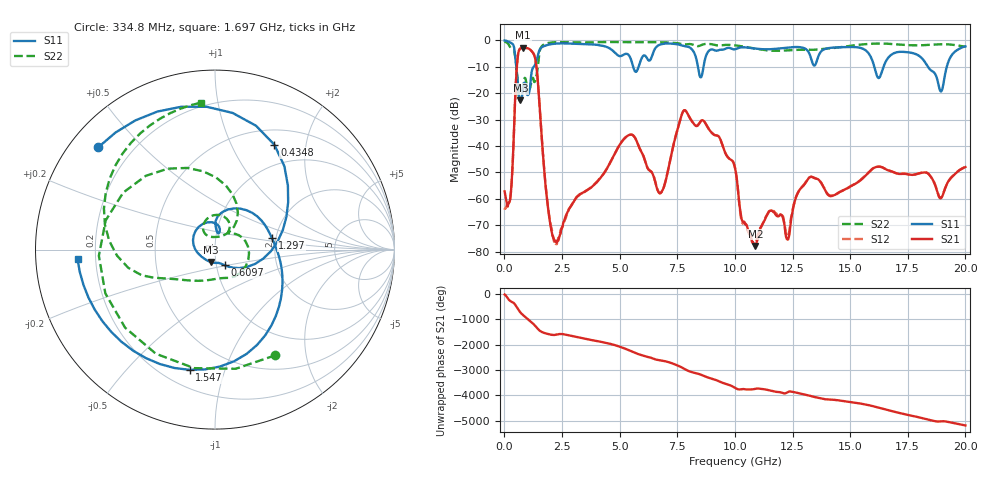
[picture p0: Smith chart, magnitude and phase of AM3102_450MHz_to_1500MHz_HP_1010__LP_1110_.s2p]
!Agilent Technologies,E8364B,MY43040894,A.07.50.67
!Agilent E8364B: A.07.50.67
!Date: Thursday, January 11, 2018 06:21:26
!Correction: S11(Full 2 Port(1,2))
!S21(Full 2 Port(1,2))
!S12(Full 2 Port(1,2))
!S22(Full 2 Port(1,2))
!S2P File: Measurements: S11, S21, S12, S22:
# Hz S  dB  R 50
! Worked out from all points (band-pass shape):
!   1601 points, 10 MHz to 20 GHz, reference 50 ohm
!   highest |S21| = -2.85 dB at 809.6 MHz (marker M1); lowest = -77.8 dB at 10.89 GHz (marker M2)
!   |S21| within 3 dB of the highest: 586 MHz to 1.303 GHz (717.5 MHz wide, 75.9 % of centre)
!   lowest |S11| = -22.7 dB at 697.2 MHz (marker M3), VSWR 1.16, Z = 47.3 - j6.61 ohm
!   |S11| at or under -10 dB: 520.8 MHz to 1.278 GHz (757.6 MHz wide, 84.2 % of centre); 16.05 GHz to 16.45 GHz (399.8 MHz wide, 2.46 % of centre); 18.37 GHz to 19.19 GHz (819.7 MHz wide, 4.36 % of centre)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
!   |S22| runs from -23.1 to -0.5 dB; largest |S21 - S12| = 0.00087
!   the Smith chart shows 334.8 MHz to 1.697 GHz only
!   S11 on the Smith chart (normalised r, x): 334.8 MHz: 0.08, +0.37; 434.8 MHz: 0.70, +1.48; 609.7 MHz: 1.10, -0.19; 1.297 GHz: 1.90, +0.27; 1.547 GHz: 0.30, -0.77; 1.697 GHz: 0.13, -0.04
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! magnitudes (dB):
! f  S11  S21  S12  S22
! 10 MHz  -0.1  -57.2  -64.1  -0.5
! 334.8 MHz  -1.3  -50.8  -51.0  -3.4
! 434.8 MHz  -3.5  -29.5  -29.6  -4.4
! 609.7 MHz  -19.7  -4.6  -4.6  -20.0
! 697.2 MHz  -22.7  -3.1  -3.1  -23.0
! 809.6 MHz  -18.2  -2.9  -2.9  -17.0
! 1.297 GHz  -9.8  -5.7  -5.7  -15.8
! 1.547 GHz  -3.3  -27.4  -27.4  -3.6
! 1.697 GHz  -2.3  -45.7  -45.7  -1.7
! 2.209 GHz  -1.3  -76.2  -76.4  -0.7
! 3.346 GHz  -1.4  -58.0  -57.9  -0.9
! 5.47 GHz  -6.8  -35.7  -35.7  -0.8
! 6.682 GHz  -1.9  -57.4  -57.3  -0.7
! 7.819 GHz  -2.2  -26.5  -26.5  -1.6
! 10.01 GHz  -3.4  -48.3  -48.3  -1.9
! 10.89 GHz  -3.1  -77.8  -77.0  -3.2
! 11.54 GHz  -3.4  -64.5  -64.4  -3.9
! 12.29 GHz  -2.7  -75.4  -74.3  -3.8
! 13.34 GHz  -7.9  -51.7  -51.7  -3.6
! 16.68 GHz  -6.4  -49.3  -49.2  -1.3
! 18.94 GHz  -19.4  -59.8  -59.7  -1.5
! 20 GHz  -2.3  -48.0  -47.9  -2.4
